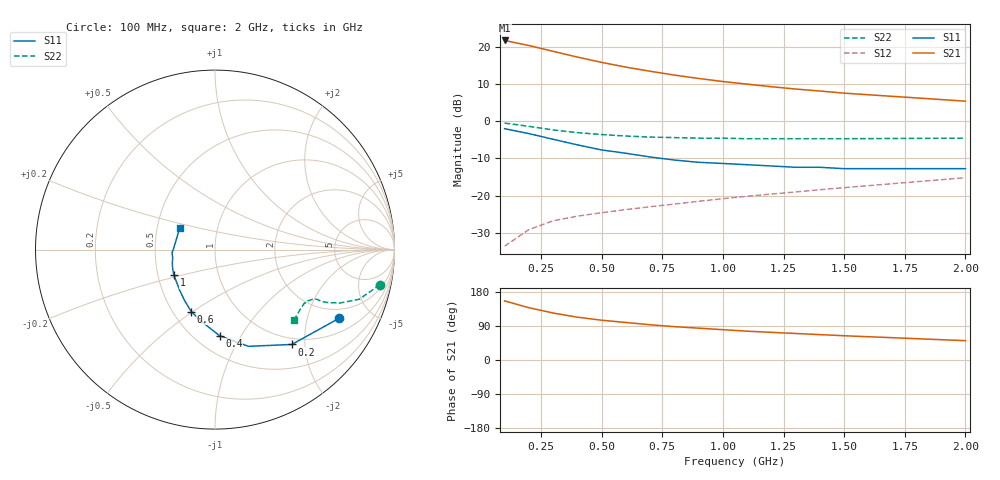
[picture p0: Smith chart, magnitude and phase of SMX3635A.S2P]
! HSMX-3635 Common Emitter
! Vce=10V Ic=5ma
# ghz s ma r 50
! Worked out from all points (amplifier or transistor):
!   16 points, 100 MHz to 2 GHz, reference 50 ohm
!   highest |S21| = 21.6 dB at 100 MHz (marker M1)
!   |S21| within 3 dB of that: start of sweep to 305.4 MHz
!   unconditionally stable (mu >= 1): 929.7 MHz to 1.912 GHz
!   at 300 MHz: K = 0.49, MSG = 22.7 dB, |S12| = -26.7 dB
!   at 900 MHz: K = 1.00, MSG = 16.5 dB, |S12| = -21.5 dB
!   at 2 GHz: K = 0.99, MSG = 10.3 dB, |S12| = -15.2 dB
!   S11 on the Smith chart (normalised r, x): 100 MHz: 1.55, -3.16; 200 MHz: 0.89, -1.74; 400 MHz: 0.65, -0.81; 600 MHz: 0.62, -0.49; 1 GHz: 0.61, -0.19; 2 GHz: 0.65, +0.16
0.1  0.79 -29.0  12.06 156.0  0.021 75.0  0.94 -12.0
0.2  0.68 -51.0  10.32 138.0  0.035 66.0  0.85 -19.0
0.3  0.57 -71.0  8.62 124.0  0.046 61.0  0.76 -23.0
0.4  0.48 -87.0  7.22 113.0  0.053 59.0  0.7 -25.0
0.5  0.41 -100.0  6.13 105.0  0.059 59.0  0.66 -26.0
0.6  0.37 -111.0  5.29 99.0  0.065 59.0  0.63 -26.0
0.7  0.33 -121.0  4.66 93.0  0.071 61.0  0.61 -27.0
0.8  0.3 -131.0  4.14 88.0  0.077 62.0  0.6 -28.0
0.9  0.28 -140.0  3.73 84.0  0.084 63.0  0.59 -29.0
1  0.27 -148.0  3.39 80.0  0.091 64.0  0.59 -30.0
1.1  0.26 -155.0  3.13 76.0  0.098 66.0  0.58 -31.0
1.2  0.25 -162.0  2.89 73.0  0.105 67.0  0.58 -32.0
1.3  0.24 -169.0  2.69 70.0  0.112 68.0  0.58 -33.0
1.4  0.24 -176.0  2.53 67.0  0.12 68.0  0.58 -34.0
1.5  0.23 178.0  2.37 64.0  0.128 69.0  0.58 -35.0
2  0.23 149.0  1.85 51.0  0.174 70.0  0.59 -42.0
